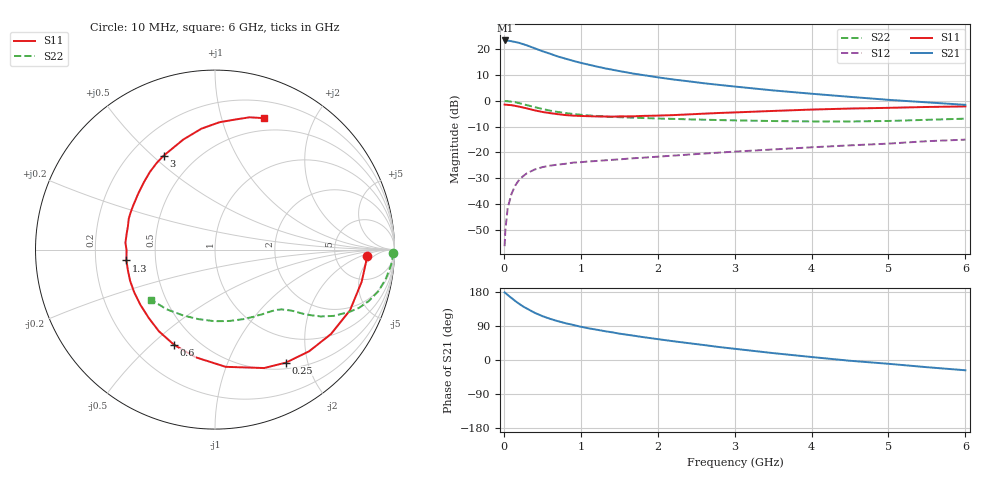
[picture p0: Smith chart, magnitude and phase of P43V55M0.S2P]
! SIEMENS Small Signal Semiconductors
! BFP182
! Si NPN RF Bipolar Junction Transistor in SOT143
! VCE = 3.5 V  IC = 5 mA
! Common Emitter S-Parameters:  March  1996
# GHz  S  MA  R  50
!  f  S11  S21  S12  S22
! GHz  MAG  ANG  MAG  ANG  MAG  ANG  MAG  ANG
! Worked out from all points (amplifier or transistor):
!   36 points, 10 MHz to 6 GHz, reference 50 ohm
!   highest |S21| = 23.5 dB at 20 MHz (marker M1)
!   |S21| within 3 dB of that: start of sweep to 397.1 MHz
!   unconditionally stable (mu >= 1): 1.598 GHz to 5.485 GHz
!   at 250 MHz: K = 0.21, MSG = 25.7 dB, |S12| = -29.3 dB
!   at 1.4 GHz: K = 0.93, MSG = 17.5 dB, |S12| = -22.9 dB
!   at 6 GHz: K = 0.95, MSG = 6.8 dB, |S12| = -15.1 dB
!   lowest NFmin = 1.20 dB at 450 MHz
!   S11 on the Smith chart (normalised r, x): 10 MHz: 11, -3; 250 MHz: 0.59, -1.65; 600 MHz: 0.37, -0.59; 1.3 GHz: 0.34, -0.05; 3 GHz: 0.33, +0.54; 6 GHz: 0.37, +1.37
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0.01  0.8465 -2.5  14.92 178.3  0.0015 79.6  0.9904 -1.0
0.02  0.844 -4.9  14.95 177.0  0.0031 88.6  0.9916 -2.0
0.05  0.8366 -12.4  14.85 171.6  0.0083 86.4  0.9848 -5.0
0.1  0.8247 -24.2  14.45 163.4  0.0157 76.5  0.9649 -9.9
0.15  0.7991 -36.1  13.93 155.5  0.0229 70.4  0.9383 -14.4
0.2  0.7721 -47.2  13.41 148.1  0.0294 65.8  0.9043 -18.4
0.25  0.7433 -57.9  12.68 141.3  0.0344 61.1  0.8659 -22.0
0.3  0.7142 -67.5  12 135.7  0.0392 56.9  0.8265 -24.8
0.4  0.6559 -84.8  10.55 124.7  0.0463 50.3  0.7572 -29.2
0.5  0.6099 -100.0  9.257 115.9  0.0515 45.0  0.6969 -32.3
0.6  0.5779 -113.1  8.27 108.7  0.0551 41.9  0.647 -34.4
0.7  0.552 -124.5  7.31 102.6  0.0577 39.3  0.6092 -36.0
0.8  0.5306 -134.0  6.624 97.2  0.0599 37.4  0.5794 -37.1
1.1  0.504 -159.8  5.071 83.7  0.0664 34.2  0.5225 -40.1
1.3  0.4973 -173.0  4.34 76.5  0.0697 33.3  0.4985 -41.9
1.7  0.5021 165.1  3.362 63.8  0.077 33.0  0.4698 -46.5
2.2  0.5291 144.0  2.61 49.6  0.0863 32.7  0.4473 -53.5
3  0.5965 118.6  1.902 29.6  0.1033 31.2  0.4181 -68.0
3.5  0.638 106.1  1.599 18.2  0.1137 29.0  0.4057 -78.7
4.5  0.71 88.0  1.198 -2.0  0.1367 24.6  0.3982 -103.4
5.5  0.7616 75.4  0.937 -19.0  0.1647 19.2  0.4288 -129.3
6  0.781 69.7  0.838 -27.1  0.1766 15.1  0.4513 -141.8
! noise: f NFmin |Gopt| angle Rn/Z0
0.45  1.2  0.27  37  0.3
0.9  1.3  0.25  75  0.23
1.8  1.9  0.21  145  0.2
